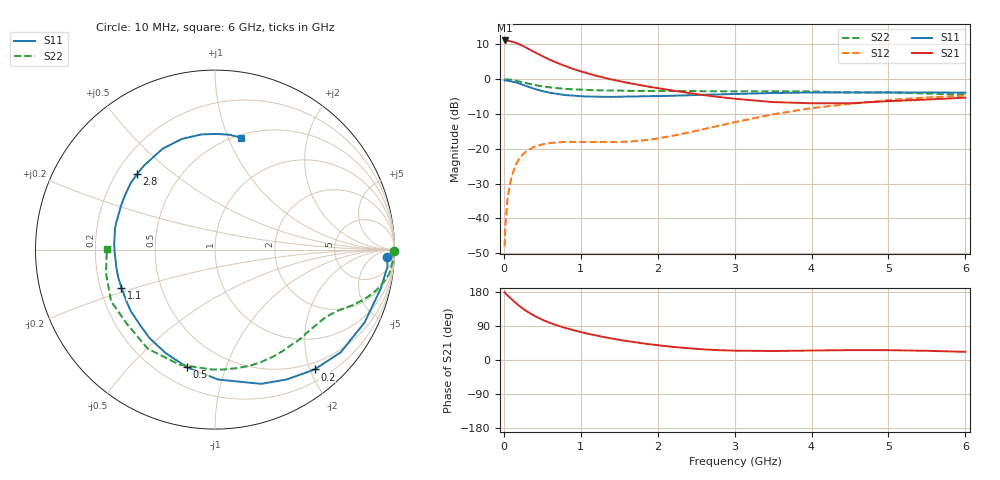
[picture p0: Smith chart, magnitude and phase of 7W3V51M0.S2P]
! Infineon Technologies  Discrete & RF Semiconductors
! BFS17W
! Si NPN RF Bipolar Junction Transistor in SOT323
! VCE = 3.5 V  IC = 1 mA
! Common Emitter S-Parameters:  August  1999
# GHz  S  MA  R  50
!  f  S11  S21  S12  S22
! GHz  MAG  ANG  MAG  ANG  MAG  ANG  MAG  ANG
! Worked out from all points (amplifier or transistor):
!   36 points, 10 MHz to 6 GHz, reference 50 ohm
!   highest |S21| = 11.1 dB at 10 MHz (marker M1)
!   |S21| within 3 dB of that: start of sweep to 369.4 MHz
!   unconditionally stable (mu >= 1): 1.033 GHz to end of sweep
!   at 250 MHz: K = 0.26, MSG = 15.5 dB, |S12| = -21.5 dB
!   at 1.4 GHz: K = 1.27, MAG = 5.8 dB, |S12| = -18.1 dB
!   at 6 GHz: K = 1.10, MAG = -2.2 dB, |S12| = -4.7 dB
!   S11 on the Smith chart (normalised r, x): 10 MHz: 22, -23; 200 MHz: 0.38, -2.07; 500 MHz: 0.31, -0.74; 1.1 GHz: 0.29, -0.18; 2.8 GHz: 0.28, +0.38; 6 GHz: 0.53, +1.11
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0.01  0.9583 -2.6  3.598 178.8  0.004 85.1  0.9999 -0.3
0.02  0.966 -5.5  3.597 176.2  0.0079 85.6  0.9962 -1.6
0.05  0.9485 -13.3  3.579 170.0  0.0205 83.4  0.9921 -4.0
0.1  0.9271 -26.0  3.462 160.8  0.0398 74.9  0.9802 -7.9
0.15  0.9044 -39.3  3.347 151.3  0.0574 67.4  0.9536 -11.2
0.2  0.8681 -50.3  3.17 142.9  0.0722 62.1  0.9274 -14.1
0.25  0.8268 -61.0  2.984 135.2  0.0837 56.2  0.8983 -16.6
0.3  0.7912 -71.0  2.792 128.3  0.0937 51.5  0.8729 -18.7
0.4  0.7241 -88.6  2.446 116.1  0.1076 44.0  0.8254 -22.1
0.5  0.6743 -103.3  2.147 106.3  0.1156 39.1  0.7888 -24.5
0.6  0.6384 -115.6  1.896 97.9  0.121 35.6  0.7626 -26.7
0.8  0.5909 -135.7  1.545 84.5  0.1253 31.8  0.7262 -31.0
1.1  0.5625 -157.9  1.206 68.9  0.1256 31.3  0.6999 -37.7
1.6  0.5629 176.2  0.889 49.9  0.1267 39.9  0.681 -50.4
2.2  0.5787 154.4  0.686 34.5  0.1544 55.5  0.6769 -67.5
2.8  0.6046 136.0  0.554 25.9  0.2148 63.2  0.6698 -85.8
3.5  0.6332 117.5  0.469 23.7  0.3128 61.6  0.6706 -107.2
4  0.6437 106.6  0.451 25.0  0.384 56.0  0.6676 -124.1
4.5  0.646 96.7  0.451 26.1  0.4419 49.4  0.6421 -139.7
5  0.6447 89.2  0.483 25.9  0.5019 42.9  0.6464 -153.6
5.5  0.6453 82.5  0.51 24.3  0.5447 36.3  0.6213 -167.9
6  0.6399 77.1  0.543 21.5  0.5841 30.1  0.6021 179.7
